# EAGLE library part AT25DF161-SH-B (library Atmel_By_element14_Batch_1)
16-megabit Minimum SPI Serial Flash Memory
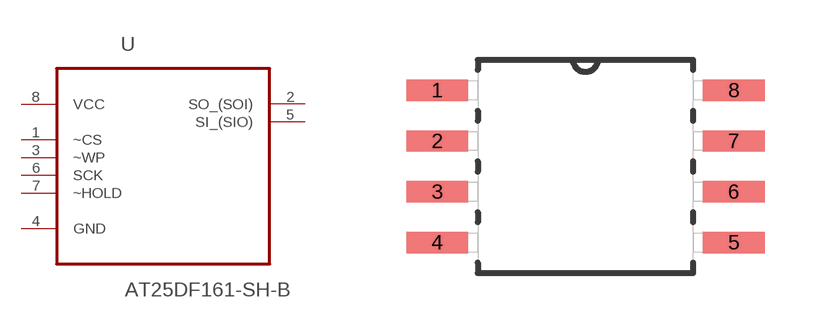
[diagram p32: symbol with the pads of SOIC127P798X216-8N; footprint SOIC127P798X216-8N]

Designator prefix U

## AT25DF161-SH-B (MPN: AT25DF161-SH-B; OC_FARNELL: 1715442; OC_NEWARK: 15R0307; PACKAGE: SOIC-8; SUPPLIER: Atmel)  [SOIC127P798X216-8N]
1  ~CS  in
2  SO_(SOI)
3  ~WP  in
4  GND  pas
5  SI_(SIO)
6  SCK  in
7  ~HOLD  in
8  VCC  pwr

## Footprint SOIC127P798X216-8N (pad centres in mm)
smd 1.549 x 0.533: 1 -3.708,1.905; 2 -3.708,0.635; 3 -3.708,-0.635; 4 -3.708,-1.905; 5 3.708,-1.905; 6 3.708,-0.635; 7 3.708,0.635; 8 3.708,1.905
